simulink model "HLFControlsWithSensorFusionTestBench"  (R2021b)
settings: Solver=ode23tb  StartTime=0.0  StopTime=scenario.StopTime  RelTol=1e-3
PostLoadFcn:
  | helperSLHLFControlsWithSensorFusionSetup
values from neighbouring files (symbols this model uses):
  vehSim3D = repmat(     struct(         'Length', 0,         'RearOverhang', 0,         'InitialPos',[0 0 0],         'InitialRot',[0 0 0]),     numVehicles,1)    [helperSLHLFControlsWithSensorFusionSetup.m]
undefined symbols (not defined in the file or in its folder): assessment, camera, Ts, v_set
libraries: drivingscenarioandsensors x8, sim3dautolib x6, simulink x4, sim3dprobsensorlib x1, sim3dlib x1, drivingsim3d x1

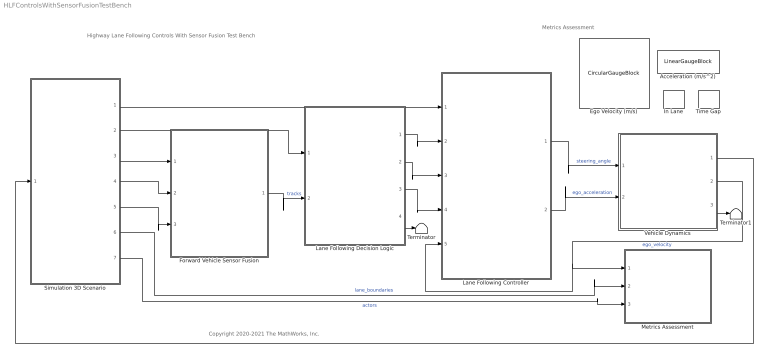
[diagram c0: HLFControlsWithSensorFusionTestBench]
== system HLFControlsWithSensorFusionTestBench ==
  note: Highway Lane Following Controls With Sensor Fusion Test Bench
  note: Metrics Assessment
  note: Copyright 2020-2021 The MathWorks, Inc.
  Acceleration (m/s^2) : LinearGaugeBlock  LabelPosition=Hide  ScaleMin=-6  ScaleMax=6
  Ego Velocity (m/s) : CircularGaugeBlock  LabelPosition=Hide  ScaleMax=50
  Forward Vehicle Sensor Fusion : ModelReference  ModelNameDialog=ForwardVehicleSensorFusion.slx  SimulationMode=Normal  CodeInterface=Top model  ModelReferenceVersion=4.3
  In Lane : LampBlock  LabelPosition=Hide
  Lane Following Controller : ModelReference  ModelNameDialog=LaneFollowingController  SimulationMode=Normal  ModelReferenceVersion=4.4
  Lane Following Decision Logic : ModelReference  ModelNameDialog=LaneFollowingDecisionLogic.slx  SimulationMode=Normal  ModelReferenceVersion=3.0
  Metrics Assessment : Subsystem
  Simulation 3D Scenario : Subsystem  VariantControl=1
  Terminator : Terminator
  Terminator1 : Terminator
  Time Gap : LampBlock  LabelPosition=Hide
  Vehicle Dynamics : Subsystem  ReferencedSubsystem=BicycleWithForceInput
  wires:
  Vehicle Dynamics/2 -> Lane Following Controller/5, Metrics Assessment/1(Longitudinal Velocity)  "ego_velocity"
  Simulation 3D Scenario/3(System Time) -> Forward Vehicle Sensor Fusion/1
  Vehicle Dynamics/1 -> Simulation 3D Scenario/1(Ego)
  Simulation 3D Scenario/6(Lane Boundaries) -> Metrics Assessment/2(Lane Boundaries_1)  "lane_boundaries"
  Simulation 3D Scenario/7(Actors) -> Metrics Assessment/3(Actors)  "actors"
  Lane Following Controller/1 -> Vehicle Dynamics/1  "steering_angle"
  Lane Following Controller/2 -> Vehicle Dynamics/2  "ego_acceleration"
  Simulation 3D Scenario/1(Set Velocity) -> Lane Following Controller/1
  Lane Following Decision Logic/1 -> Lane Following Controller/2
  Lane Following Decision Logic/3 -> Lane Following Controller/4
  Lane Following Decision Logic/2 -> Lane Following Controller/3
  Simulation 3D Scenario/4(Vision Detections) -> Forward Vehicle Sensor Fusion/2
  Simulation 3D Scenario/5(Radar Detections) -> Forward Vehicle Sensor Fusion/3
  Forward Vehicle Sensor Fusion/1 -> Lane Following Decision Logic/2  "tracks"
  Simulation 3D Scenario/2(Lanes) -> Lane Following Decision Logic/1
  Lane Following Decision Logic/4 -> Terminator/1
  Vehicle Dynamics/3 -> Terminator1/1

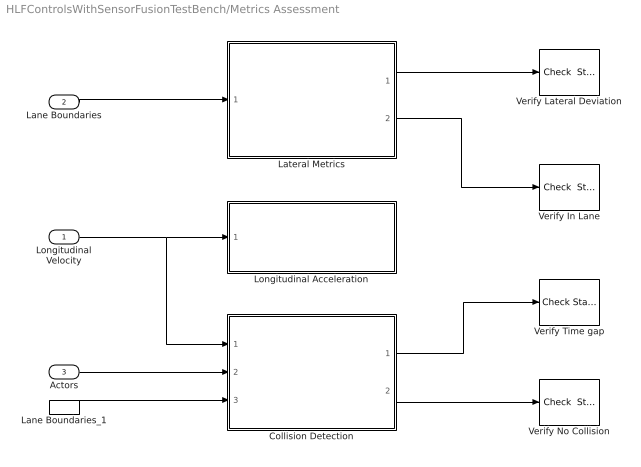
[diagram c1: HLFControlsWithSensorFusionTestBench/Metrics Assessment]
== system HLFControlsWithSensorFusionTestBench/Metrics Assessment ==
  Longitudinal Velocity : Inport
  Lane Boundaries : Inport  Port=2
  Actors : Inport  Port=3
  Collision Detection : Subsystem  ReferencedSubsystem=CollisionDetection
  Lane Boundaries_1 : InportShadow  Port=2
  Lateral Metrics : Subsystem  ReferencedSubsystem=LateralMetrics
  Longitudinal Acceleration : Subsystem
  Verify In Lane : simulink/Model Verification/Check  Static Range  Description=1 <= u <= 1  max=1  max_included=on  min=1  min_included=on  enabled=on  stopWhenAssertionFail=on  export=off  icon=graphic
  Verify Lateral Deviation : simulink/Model Verification/Check  Static Range  Description=-assessment.LateralDeviationMax <= u <= assessment.LateralDeviationMax  max=assessment.LateralDeviationMax  max_included=on  min=-assessment.LateralDeviationMax  min_included=on  enabled=on  stopWhenAssertionFail=on  export=off  icon=graphic
  Verify No Collision : simulink/Model Verification/Check  Static Range  Description=0 <= u <= 0  max=0  max_included=on  min=0  min_included=on  enabled=on  stopWhenAssertionFail=on  export=off  icon=graphic
  Verify Time gap : simulink/Model Verification/Check Static  Lower Bound  Description=assessment.TimeGap <= u  min=assessment.TimeGap  min_included=on  enabled=on  stopWhenAssertionFail=off  export=off  icon=graphic
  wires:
  Lane Boundaries/1 -> Lateral Metrics/1
  Collision Detection/1 -> Verify Time gap/1
  Lateral Metrics/1 -> Verify Lateral Deviation/1
  Collision Detection/2 -> Verify No Collision/1
  Longitudinal Velocity/1 -> Collision Detection/1, Longitudinal Acceleration/1(Longitudinal Velocity)
  Actors/1 -> Collision Detection/2
  Lateral Metrics/2 -> Verify In Lane/1
  Lane Boundaries_1/1 -> Collision Detection/3

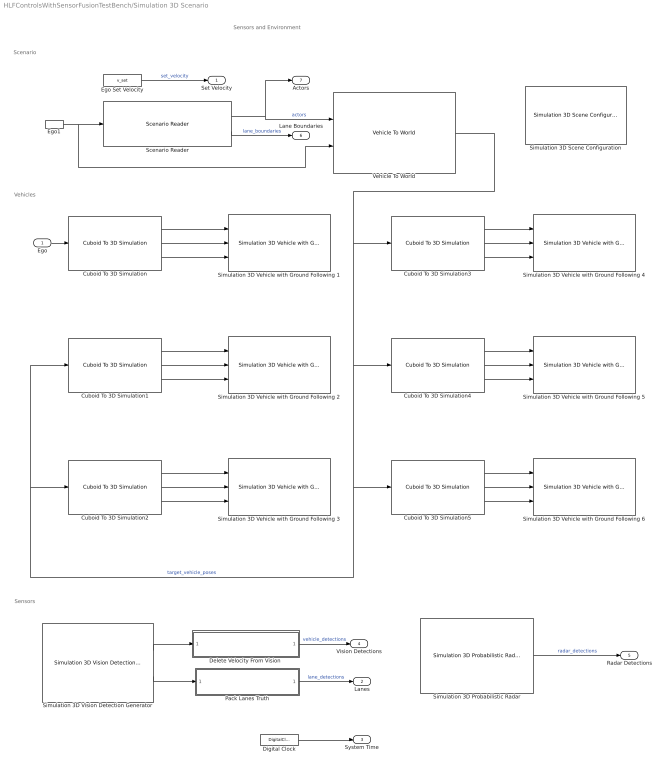
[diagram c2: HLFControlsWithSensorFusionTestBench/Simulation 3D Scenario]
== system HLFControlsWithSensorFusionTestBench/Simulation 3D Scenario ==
  note: Scenario
  note: Vehicles
  note: Sensors and Environment
  note: Sensors
  Ego : Inport
  Cuboid To 3D Simulation : drivingscenarioandsensors/Cuboid To 3D Simulation  SpecifyActorID=off  ActorIDToConvert=1  SimulateUsing=Interpreted execution
  Cuboid To 3D Simulation1 : drivingscenarioandsensors/Cuboid To 3D Simulation  SpecifyActorID=on  ActorIDToConvert=2  SimulateUsing=Interpreted execution
  Cuboid To 3D Simulation2 : drivingscenarioandsensors/Cuboid To 3D Simulation  SpecifyActorID=on  ActorIDToConvert=3  SimulateUsing=Interpreted execution
  Cuboid To 3D Simulation3 : drivingscenarioandsensors/Cuboid To 3D Simulation  SpecifyActorID=on  ActorIDToConvert=4  SimulateUsing=Interpreted execution
  Cuboid To 3D Simulation4 : drivingscenarioandsensors/Cuboid To 3D Simulation  SpecifyActorID=on  ActorIDToConvert=5  SimulateUsing=Interpreted execution
  Cuboid To 3D Simulation5 : drivingscenarioandsensors/Cuboid To 3D Simulation  SpecifyActorID=on  ActorIDToConvert=6  SimulateUsing=Interpreted execution
  "Delete Velocity From Vision " : MATLAB Function  TreatAsAtomicUnit=on  mask(Pack vision detections){structInit=Simulink.Bus.createMATLABStruct('BusVision'), measurementNoise=camera.MeasurementNoise}
      mask prompts: structInit "Output struct"; measurementNoise "Measurement noise"
      mask help: Packs vision detections to match bus used by vision processing algorithm. This includes replacing the measurement noise and disabling the velocity measurement.
  Digital Clock : DigitalClock  SampleTime=Ts
  Ego Set Velocity : Constant  Value=v_set  SampleTime=Ts
  Ego1 : InportShadow
  Pack Lanes Truth : MATLAB Function  TreatAsAtomicUnit=on  mask{structObj=Simulink.Bus.createMATLABStruct('LaneSensor')}
      mask prompts: structObj "Output struct"
  Scenario Reader : drivingscenarioandsensors/Scenario Reader  ScenarioSource=From workspace  ScenarioFileName=dblLaneChangeDrivingScenario.mat  ScenarioVariableName=scenario  OutputCoordinateSystem=Vehicle coordinates  EgoVehicleSource=Input port  EgoVehicleActorID=1  OrientVehiclesOnRoad=off  OutputEgoVehiclePose=off  OutputEgoVehicleState=off  SampleTime=0.1  LaneBoundaryOutput=Ego vehicle lane boundaries  LaneBoundaryDistance=0:0.5:70  LaneBoundaryLocation=Center of lane markings  BusNameSource=Auto  BusName=BusActors  BusNumActorsSource=Scenario  BusNumActors=100  BusName2Source=Auto  BusName2=BusLaneBoundaries  BusNumLaneBoundariesSource=Scenario  BusNumLaneBoundaries=10  BusName3Source=Auto  BusName3=BusEgoActor  BusName4Source=Auto  BusName4=BusEgoState  ShowCoordinateLabels=on  SimulateUsing=Interpreted execution
  Simulation 3D Probabilistic Radar : sim3dprobsensorlib/Simulation 3D Probabilistic Radar  Priority=1  sensorTag=Sim3dSensor2  sensorId=2  sensorName=Sim3dSensor2  vehTagList={'Scene Origin';'SimulinkVehicle1';'SimulinkVehicle4';'SimulinkVehicle5';'SimulinkVehicle6';'vehSim3D(2).InitialRot';'vehSim3D(3).InitialRot'}  vehTag=SimulinkVehicle1  mountLoc=Origin  offsetFlag=on  tmountOffset=radar.PositionSim3d  rmountOffset=radar.Rotation  AzimuthResolution=0.8  ElevationResolution=8  RangeResolution=1  RangeRateResolution=1  AzimuthBiasFraction=0.1  ElevationBiasFraction=0.1  RangeBiasFraction=0.05  RangeRateBiasFraction=0.05  FieldOfView=radar.FieldOfView  DetectionRange=radar.DetectionRanges  RangeRateLimits=[ -100, 100 ]  DetectionProbability=0.9  FalseAlarmRate=1e-6  ReferenceRange=150  ReferenceRCS=0  HasElevation=off  HasRangeRate=on  HasNoise=off  HasFalseAlarms=off  InitialSeedSource=Repeatable  InitialSeed=0  MaxNumDetections=50  DetectionCoordinates=Sensor spherical  SpecifyOutputBusName=off  BusName=BusSimulation3DRadarTruthSensor  SampleTime=-1  mountPoint=[2.424 0 0.8]  mountOrientation=[0 0 0]  aMode=3  ID=2
  Simulation 3D Scene Configuration : sim3dlib/Simulation 3D Scene Configuration  Priority=0  ProjectFormat_internal=Default Scenes  ProjectFormat=Default Scenes  SceneDesc=Curved road  ProjectName=/mathworks/devel/bat/BR2021bd/build/matlab/toolbox/shared/sim3d_projects/automotive_project/UE4/LinuxNoEditor/AutoVrtlEnv.sh  ScenePath=/Game/Maps/HwStrght  vehTagList={'Scene Origin';'SimulinkVehicle1';'SimulinkVehicle4';'SimulinkVehicle5';'SimulinkVehicle6';'vehSim3D(2).InitialRot';'vehSim3D(3).InitialRot'}  vehTag=SimulinkVehicle1  OpVisEn=off  Ts=0.1  EnableWindow=on  EnableWeather=off  SunAltitude=40.0  SunAzimuth=90  clouds=10  wind=1  fog=0  rain=0  sensorTag=MainCamera1  sensorId=1  sensorName=MainCamera1  mountLoc=Origin  offsetFlag=off  tmountOffset=[0, 0, 0]  rmountOffset=[0, 0, 0]  HorizontalResolution=1280  VerticalResolution=720  HorizontalFOV=60  mountPoint=[0 0 0]  mountOrientation=[0 0 0]  aMode=3  ID=1
  Simulation 3D Vehicle with Ground Following 1 : sim3dautolib/Simulation 3D Vehicle with Ground Following  Priority=-1  PassVehMesh=Sedan  PassVehMesh_Internal=Sedan  MeshPath=/MathWorksSimulation/Vehicles/Muscle/Meshes/SK_MuscleCar.SK_MuscleCar  TrackWidth=1.9  WheelBase=3  WheelRadius=0.35  VehColor=Blue  VehColor_Internal=Blue  InitialPos=vehSim3D(1).InitialPos  InitialRot=vehSim3D(1).InitialRot  ActorName=SimulinkVehicle1  SampleTime=-1  ActorType=SimulinkVehicle  ID=1  aMode=3  ActorTag=SimulinkVehicle1  CoordinateScheme=ISO  VehLightsControl=off  HeadlightColor=[ 1, 1, 1 ]  HighBeamIntensity=100000  LowBeamIntensity=60000  HighBeamConeAngle=70  LowBeamConeAngle=70  LeftHeadlightOrientation=[ 0, 0 ]  RightHeadlightOrientation=[ 0, 0 ]  BrakelightIntensity=500  ReverselightIntensity=500  SignallightIntensity=500  SignallightPeriod=1  SignalPulseWidth=50  TransformOutportEnabled=off
  Simulation 3D Vehicle with Ground Following 2 : sim3dautolib/Simulation 3D Vehicle with Ground Following  Priority=-1  PassVehMesh=Sedan  PassVehMesh_Internal=Sedan  MeshPath=/MathWorksSimulation/Vehicles/Muscle/Meshes/SK_MuscleCar.SK_MuscleCar  TrackWidth=1.9  WheelBase=3  WheelRadius=0.35  VehColor=Red  VehColor_Internal=Red  InitialPos=vehSim3D(2).InitialPos  InitialRot=vehSim3D(2).InitialRot  ActorName=vehSim3D(2).InitialRot  SampleTime=-1  ActorType=SimulinkVehicle  ID=C  aMode=3  ActorTag=vehSim3D(2).InitialRot  CoordinateScheme=ISO  VehLightsControl=off  HeadlightColor=[ 1, 1, 1 ]  HighBeamIntensity=100000  LowBeamIntensity=60000  HighBeamConeAngle=70  LowBeamConeAngle=70  LeftHeadlightOrientation=[ 0, 0 ]  RightHeadlightOrientation=[ 0, 0 ]  BrakelightIntensity=500  ReverselightIntensity=500  SignallightIntensity=500  SignallightPeriod=1  SignalPulseWidth=50  TransformOutportEnabled=off
  Simulation 3D Vehicle with Ground Following 3 : sim3dautolib/Simulation 3D Vehicle with Ground Following  Priority=-1  PassVehMesh=Muscle car  PassVehMesh_Internal=Muscle car  MeshPath=/MathWorksSimulation/Vehicles/Muscle/Meshes/SK_MuscleCar.SK_MuscleCar  TrackWidth=1.9  WheelBase=3  WheelRadius=0.35  VehColor=Black  VehColor_Internal=Black  InitialPos=vehSim3D(3).InitialPos  InitialRot=vehSim3D(3).InitialRot  ActorName=vehSim3D(3).InitialRot  SampleTime=-1  ActorType=SimulinkVehicle  ID=C  aMode=3  ActorTag=vehSim3D(3).InitialRot  CoordinateScheme=ISO  VehLightsControl=off  HeadlightColor=[ 1, 1, 1 ]  HighBeamIntensity=100000  LowBeamIntensity=60000  HighBeamConeAngle=70  LowBeamConeAngle=70  LeftHeadlightOrientation=[ 0, 0 ]  RightHeadlightOrientation=[ 0, 0 ]  BrakelightIntensity=500  ReverselightIntensity=500  SignallightIntensity=500  SignallightPeriod=1  SignalPulseWidth=50  TransformOutportEnabled=off
  Simulation 3D Vehicle with Ground Following 4 : sim3dautolib/Simulation 3D Vehicle with Ground Following  Priority=-1  PassVehMesh=Hatchback  PassVehMesh_Internal=Hatchback  MeshPath=/MathWorksSimulation/Vehicles/Muscle/Meshes/SK_MuscleCar.SK_MuscleCar  TrackWidth=1.9  WheelBase=3  WheelRadius=0.35  VehColor=Orange  VehColor_Internal=Orange  InitialPos=vehSim3D(4).InitialPos  InitialRot=vehSim3D(4).InitialRot  ActorName=SimulinkVehicle4  SampleTime=-1  ActorType=SimulinkVehicle  ID=4  aMode=3  ActorTag=SimulinkVehicle4  CoordinateScheme=ISO  VehLightsControl=off  HeadlightColor=[ 1, 1, 1 ]  HighBeamIntensity=100000  LowBeamIntensity=60000  HighBeamConeAngle=70  LowBeamConeAngle=70  LeftHeadlightOrientation=[ 0, 0 ]  RightHeadlightOrientation=[ 0, 0 ]  BrakelightIntensity=500  ReverselightIntensity=500  SignallightIntensity=500  SignallightPeriod=1  SignalPulseWidth=50  TransformOutportEnabled=off
  Simulation 3D Vehicle with Ground Following 5 : sim3dautolib/Simulation 3D Vehicle with Ground Following  Priority=-1  PassVehMesh=Small pickup truck  PassVehMesh_Internal=Small pickup truck  MeshPath=/MathWorksSimulation/Vehicles/Muscle/Meshes/SK_MuscleCar.SK_MuscleCar  TrackWidth=1.9  WheelBase=3  WheelRadius=0.35  VehColor=Green  VehColor_Internal=Green  InitialPos=vehSim3D(5).InitialPos  InitialRot=vehSim3D(5).InitialRot  ActorName=SimulinkVehicle5  SampleTime=-1  ActorType=SimulinkVehicle  ID=5  aMode=3  ActorTag=SimulinkVehicle5  CoordinateScheme=ISO  VehLightsControl=off  HeadlightColor=[ 1, 1, 1 ]  HighBeamIntensity=100000  LowBeamIntensity=60000  HighBeamConeAngle=70  LowBeamConeAngle=70  LeftHeadlightOrientation=[ 0, 0 ]  RightHeadlightOrientation=[ 0, 0 ]  BrakelightIntensity=500  ReverselightIntensity=500  SignallightIntensity=500  SignallightPeriod=1  SignalPulseWidth=50  TransformOutportEnabled=off
  Simulation 3D Vehicle with Ground Following 6 : sim3dautolib/Simulation 3D Vehicle with Ground Following  Priority=-1  PassVehMesh=Sport utility vehicle  PassVehMesh_Internal=Sport utility vehicle  MeshPath=/MathWorksSimulation/Vehicles/Muscle/Meshes/SK_MuscleCar.SK_MuscleCar  TrackWidth=1.9  WheelBase=3  WheelRadius=0.35  VehColor=Blue  VehColor_Internal=Blue  InitialPos=vehSim3D(6).InitialPos  InitialRot=vehSim3D(6).InitialRot  ActorName=SimulinkVehicle6  SampleTime=-1  ActorType=SimulinkVehicle  ID=6  aMode=3  ActorTag=SimulinkVehicle6  CoordinateScheme=ISO  VehLightsControl=off  HeadlightColor=[ 1, 1, 1 ]  HighBeamIntensity=100000  LowBeamIntensity=60000  HighBeamConeAngle=70  LowBeamConeAngle=70  LeftHeadlightOrientation=[ 0, 0 ]  RightHeadlightOrientation=[ 0, 0 ]  BrakelightIntensity=500  ReverselightIntensity=500  SignallightIntensity=500  SignallightPeriod=1  SignalPulseWidth=50  TransformOutportEnabled=off
  Simulation 3D Vision Detection Generator : drivingsim3d/Simulation 3D Vision Detection Generator  Priority=1  sensorTag=Sim3dSensor255  sensorId=1  sensorName=Sim3dSensor1  vehTagList={'Scene Origin';'SimulinkVehicle1';'SimulinkVehicle4';'SimulinkVehicle5';'SimulinkVehicle6';'vehSim3D(2).InitialRot';'vehSim3D(3).InitialRot'}  vehTag=SimulinkVehicle1  mountLoc=Origin  offsetFlag=on  tmountOffset=camera.PositionSim3d  rmountOffset=camera.Rotation  DetectorOutput=Objects only  MaxNumDetections=20  MaxNumLanes=30  laneSampleDistances=0:0.5:9.5  BusNameSource=Property  BusName=BusObjectDetections  BusName2Source=Property  BusName2=BusLaneDetections  MaxRange=camera.DetectionRanges(2)  BoundingBoxAccuracy=5  ProcessNoiseIntensity=5  MaxSpeed=50  MaxAllowedOcclusion=0.5  MinObjectImageSize=camera.MinObjectImageSize  DetectionProbability=1  FalsePositivesPerImage=0  MinLaneImageSize=[ 20, 3 ]  LaneBoundaryAccuracy=3  HasNoise=off  InitialSeedSource=Repeatable  InitialSeed=1  uniqueActorIdentifier=[]  actorClassInteger=0  cuboidLength=4.7  cuboidWidth=1.8  cuboidHeight=1.4  rotationalCenter={[-1.35, 0, 0]}  focalLength=camera.FocalLength  opticalCenter=camera.PrincipalPoint  imageSize=camera.ImageSize  radialDistortionCoefficients=[0, 0]  tangentialDistortionCoefficients=[0, 0]  cameraAxisSkew=0  actorTruthOutportEnabled=off  laneTruthOutportEnabled=on  SampleTime=-1  checkedSampleTime=0.1  mountPoint=[0.57 0 1.2]  mountOrientation=[0 0 0]  aMode=3  ID=1
  Vehicle To World : drivingscenarioandsensors/Vehicle To World  BusNameSource=Auto  BusName=BusVehicleToWorldActors  SimulateUsing=Interpreted execution
  Set Velocity : Outport  Unit=m/s  VectorParamsAs1DForOutWhenUnconnected=off
  Lanes : Outport  Port=2
  System Time : Outport  Port=3  VectorParamsAs1DForOutWhenUnconnected=off
  Vision Detections : Outport  Port=4  OutDataTypeStr=Bus: BusVision
  Radar Detections : Outport  Port=5
  Lane Boundaries : Outport  Port=6
  Actors : Outport  Port=7
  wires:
  Cuboid To 3D Simulation/2 -> Simulation 3D Vehicle with Ground Following 1/2
  Cuboid To 3D Simulation/1 -> Simulation 3D Vehicle with Ground Following 1/1
  Cuboid To 3D Simulation/3 -> Simulation 3D Vehicle with Ground Following 1/3
  Ego/1 -> Cuboid To 3D Simulation/1
  Cuboid To 3D Simulation1/2 -> Simulation 3D Vehicle with Ground Following 2/2
  Cuboid To 3D Simulation1/1 -> Simulation 3D Vehicle with Ground Following 2/1
  Cuboid To 3D Simulation1/3 -> Simulation 3D Vehicle with Ground Following 2/3
  Scenario Reader/1 -> Vehicle To World/1, Actors/1  "actors"
  Vehicle To World/1 -> Cuboid To 3D Simulation3/1, Cuboid To 3D Simulation4/1, Cuboid To 3D Simulation5/1, Cuboid To 3D Simulation2/1, Cuboid To 3D Simulation1/1  "target_vehicle_poses"
  Cuboid To 3D Simulation3/2 -> Simulation 3D Vehicle with Ground Following 4/2
  Cuboid To 3D Simulation3/3 -> Simulation 3D Vehicle with Ground Following 4/3
  Cuboid To 3D Simulation2/2 -> Simulation 3D Vehicle with Ground Following 3/2
  Cuboid To 3D Simulation3/1 -> Simulation 3D Vehicle with Ground Following 4/1
  Cuboid To 3D Simulation2/3 -> Simulation 3D Vehicle with Ground Following 3/3
  Cuboid To 3D Simulation2/1 -> Simulation 3D Vehicle with Ground Following 3/1
  Cuboid To 3D Simulation4/3 -> Simulation 3D Vehicle with Ground Following 5/3
  Cuboid To 3D Simulation5/2 -> Simulation 3D Vehicle with Ground Following 6/2
  Cuboid To 3D Simulation5/3 -> Simulation 3D Vehicle with Ground Following 6/3
  Cuboid To 3D Simulation5/1 -> Simulation 3D Vehicle with Ground Following 6/1
  Cuboid To 3D Simulation4/2 -> Simulation 3D Vehicle with Ground Following 5/2
  Cuboid To 3D Simulation4/1 -> Simulation 3D Vehicle with Ground Following 5/1
  Scenario Reader/2 -> Lane Boundaries/1  "lane_boundaries"
  Ego1/1 -> Vehicle To World/2, Scenario Reader/1
  Ego Set Velocity/1 -> Set Velocity/1  "set_velocity"
  Simulation 3D Vision Detection Generator/1 -> "Delete Velocity From Vision "/1(detections)
  Simulation 3D Probabilistic Radar/1 -> Radar Detections/1  "radar_detections"
  "Delete Velocity From Vision "/1(updatedDetections) -> Vision Detections/1  "vehicle_detections"
  Digital Clock/1 -> System Time/1
  Simulation 3D Vision Detection Generator/2 -> Pack Lanes Truth/1(lanesTruth)
  Pack Lanes Truth/1(lanes) -> Lanes/1  "lane_detections"

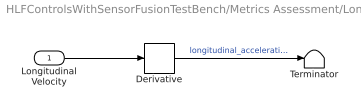
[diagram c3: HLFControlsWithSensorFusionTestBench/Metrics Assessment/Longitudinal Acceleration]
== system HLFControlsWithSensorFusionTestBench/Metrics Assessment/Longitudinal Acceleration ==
  Longitudinal Velocity : Inport
  Derivative : Derivative
  Terminator : Terminator
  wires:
  Derivative/1 -> Terminator/1  "longitudinal_acceleration"
  Longitudinal Velocity/1 -> Derivative/1

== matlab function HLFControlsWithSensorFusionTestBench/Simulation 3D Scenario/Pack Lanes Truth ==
function lanes = packLanesTruth(lanesTruth, structObj)
% Assign lane parameters from ground-truth lane boundaries.

% Assign lanes struct object to output variable
lanes = structObj;

% Find ego-vehicle lane boundary indices
lbNum = [1, 1];
for j = 1:length(lanesTruth.LaneBoundaries)-1
    yleftLane = lanesTruth.LaneBoundaries(j+1).Coordinates(1,2);
    yrightLane = lanesTruth.LaneBoundaries(j).Coordinates(1,2);
    
    if ((0 >= yleftLane) && (0 <= yrightLane))
        lbNum(1) = j;
        lbNum(2) = j+1;
        break;
    elseif ((0 >= yrightLane) && (0 <= yleftLane))
        lbNum(1) = j+1;
        lbNum(2) = j;
        break;
    end
end

%% Pack left lane info
leftLaneCoordinates = lanesTruth.LaneBoundaries(lbNum(1)).Coordinates;
% Get parabolic lane boundary parameters using polyfit for the left lane.
leftLaneParameters = polyfit(leftLaneCoordinates(:,1),...
    leftLaneCoordinates(:,2),2);

% Assign lane parameters to output bus, lanes.
lanes.Left.Curvature = single(2 * leftLaneParameters(1));
lanes.Left.HeadingAngle = single(leftLaneParameters(2));
lanes.Left.LateralOffset = single(leftLaneParameters(3));

lanes.Left.Strength = single(lanesTruth.LaneBoundaries(lbNum(1)).Strength);


%% Pack right lane info
rightLaneCoordinates = lanesTruth.LaneBoundaries(lbNum(2)).Coordinates;
% Get parabolic lane boundary parameters using polyfit for the right lane
rightLaneParameters = polyfit(rightLaneCoordinates(:,1),...
    rightLaneCoordinates(:,2),2);

% Assign lane parameters to output bus, lanes.
lanes.Right.Curvature = single(2 * rightLaneParameters(1));
lanes.Right.HeadingAngle = single(rightLaneParameters(2));
lanes.Right.LateralOffset = single(rightLaneParameters(3));

lanes.Right.Strength = single(lanesTruth.LaneBoundaries(lbNum(2)).Strength);

end

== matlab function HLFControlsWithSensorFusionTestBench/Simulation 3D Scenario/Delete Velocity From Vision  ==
function updatedDetections = deleteVelocityFromVision(detections,structInit,measurementNoise)

updatedDetections = structInit;
updatedDetections.NumDetections = detections.NumDetections;
updatedDetections.IsValidTime = detections.IsValidTime;
for n = 1:detections.NumDetections
    updatedDetections.Detections(n).Time = detections.Detections(n).Time;
    updatedDetections.Detections(n).Measurement = detections.Detections(n).Measurement(1:3);
    updatedDetections.Detections(n).MeasurementNoise = measurementNoise;
    updatedDetections.Detections(n).SensorIndex = detections.Detections(n).SensorIndex;
    updatedDetections.Detections(n).ObjectClassID = detections.Detections(n).ObjectClassID;
    updatedDetections.Detections(n).ObjectAttributes = detections.Detections(n).ObjectAttributes;
    updatedDetections.Detections(n).MeasurementParameters = detections.Detections(n).MeasurementParameters;
    updatedDetections.Detections(n).MeasurementParameters.HasVelocity = false;
end
